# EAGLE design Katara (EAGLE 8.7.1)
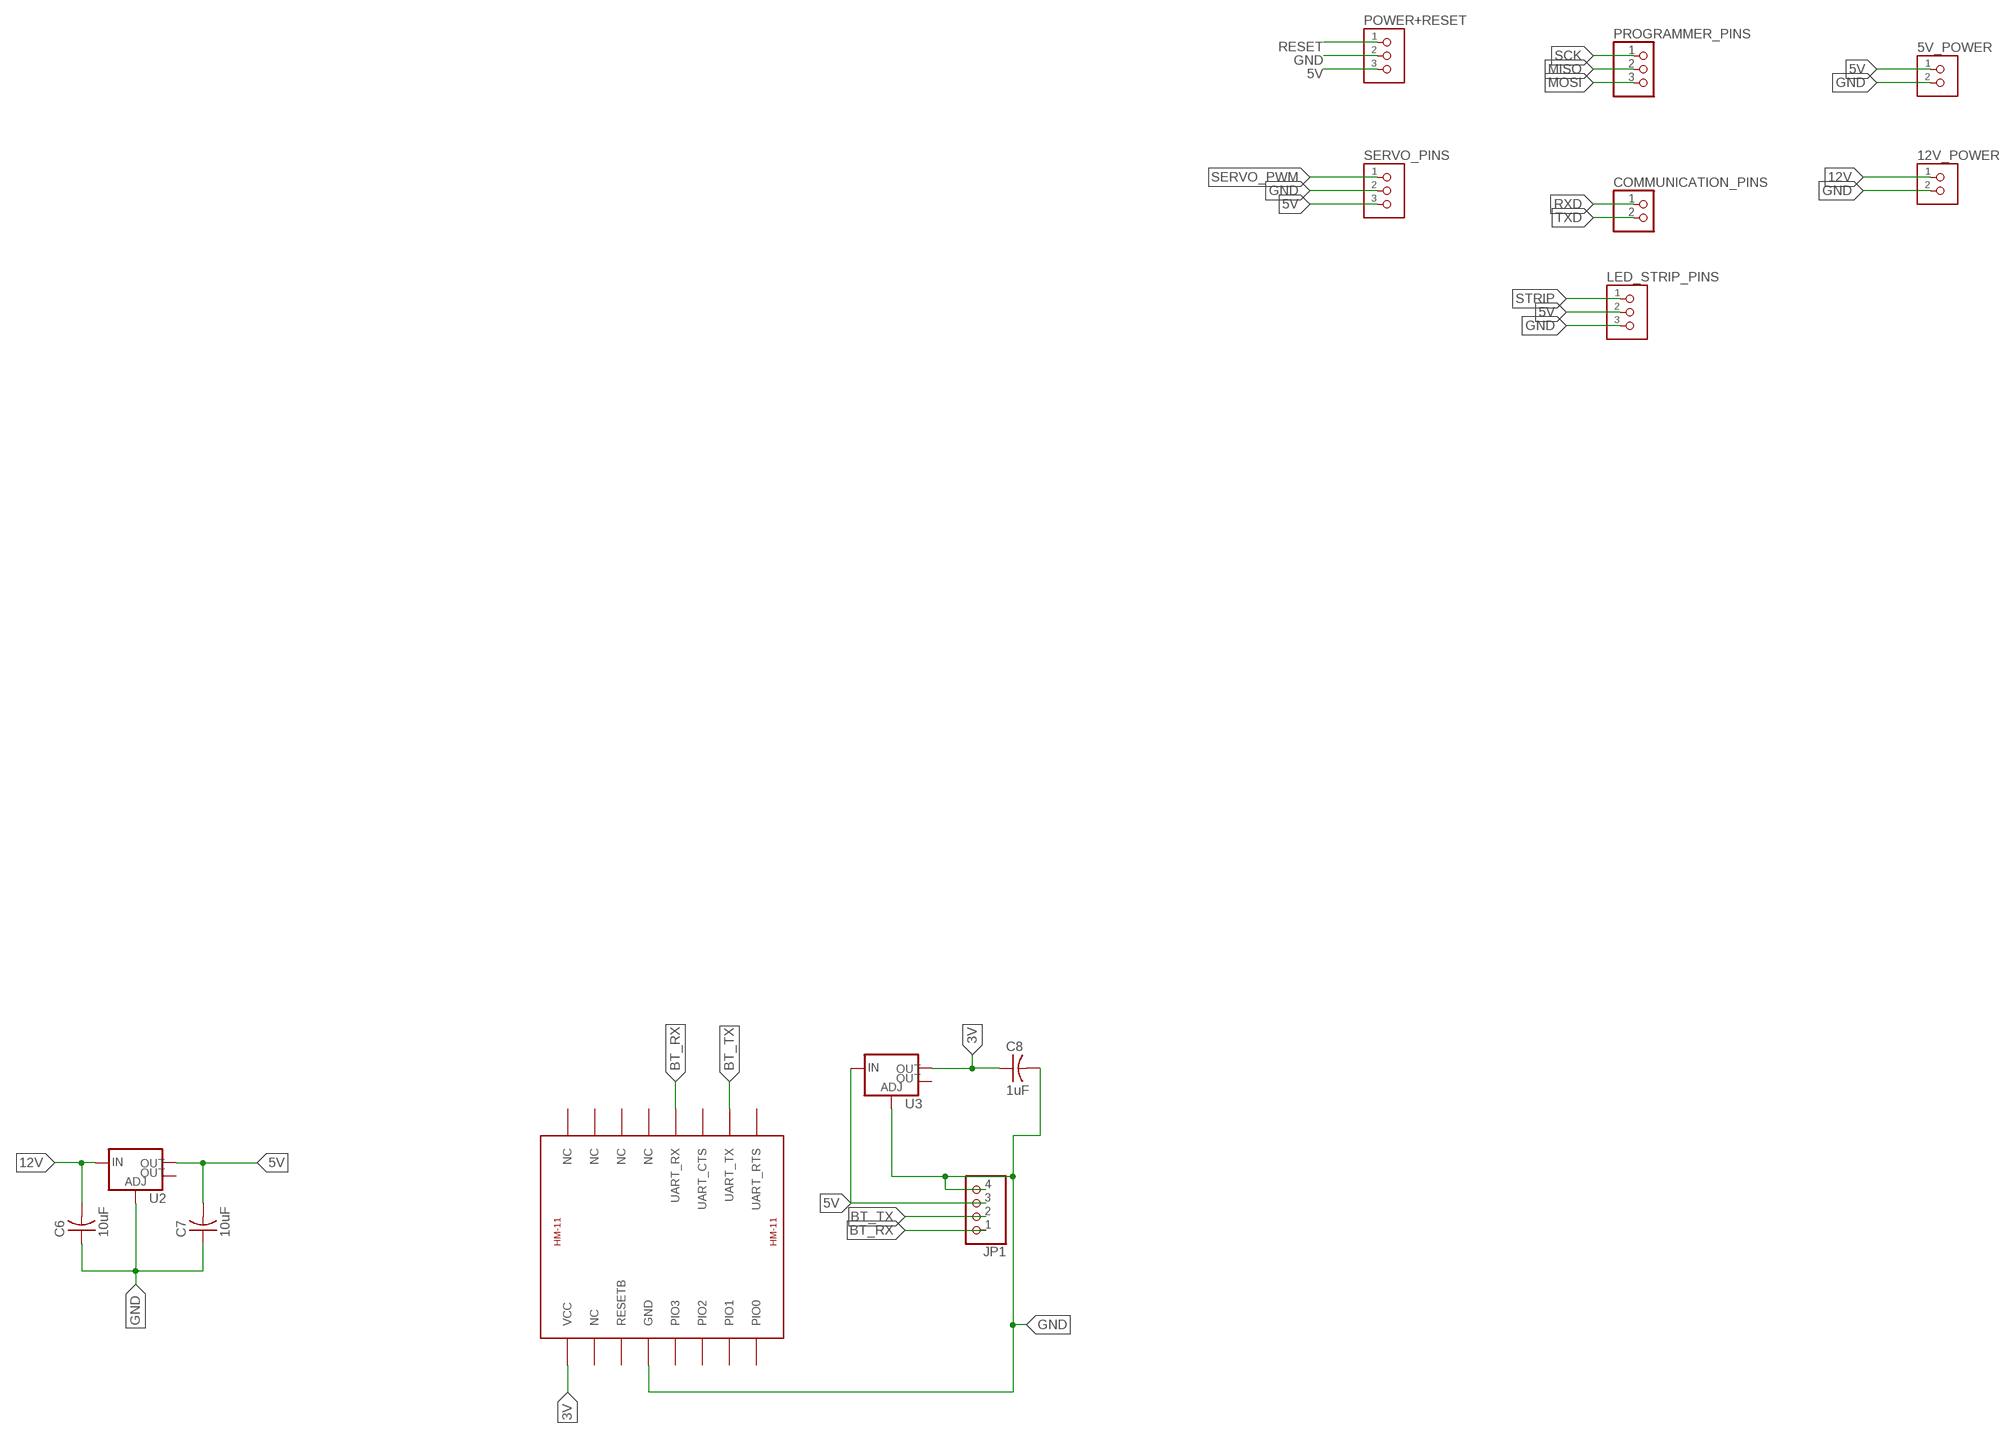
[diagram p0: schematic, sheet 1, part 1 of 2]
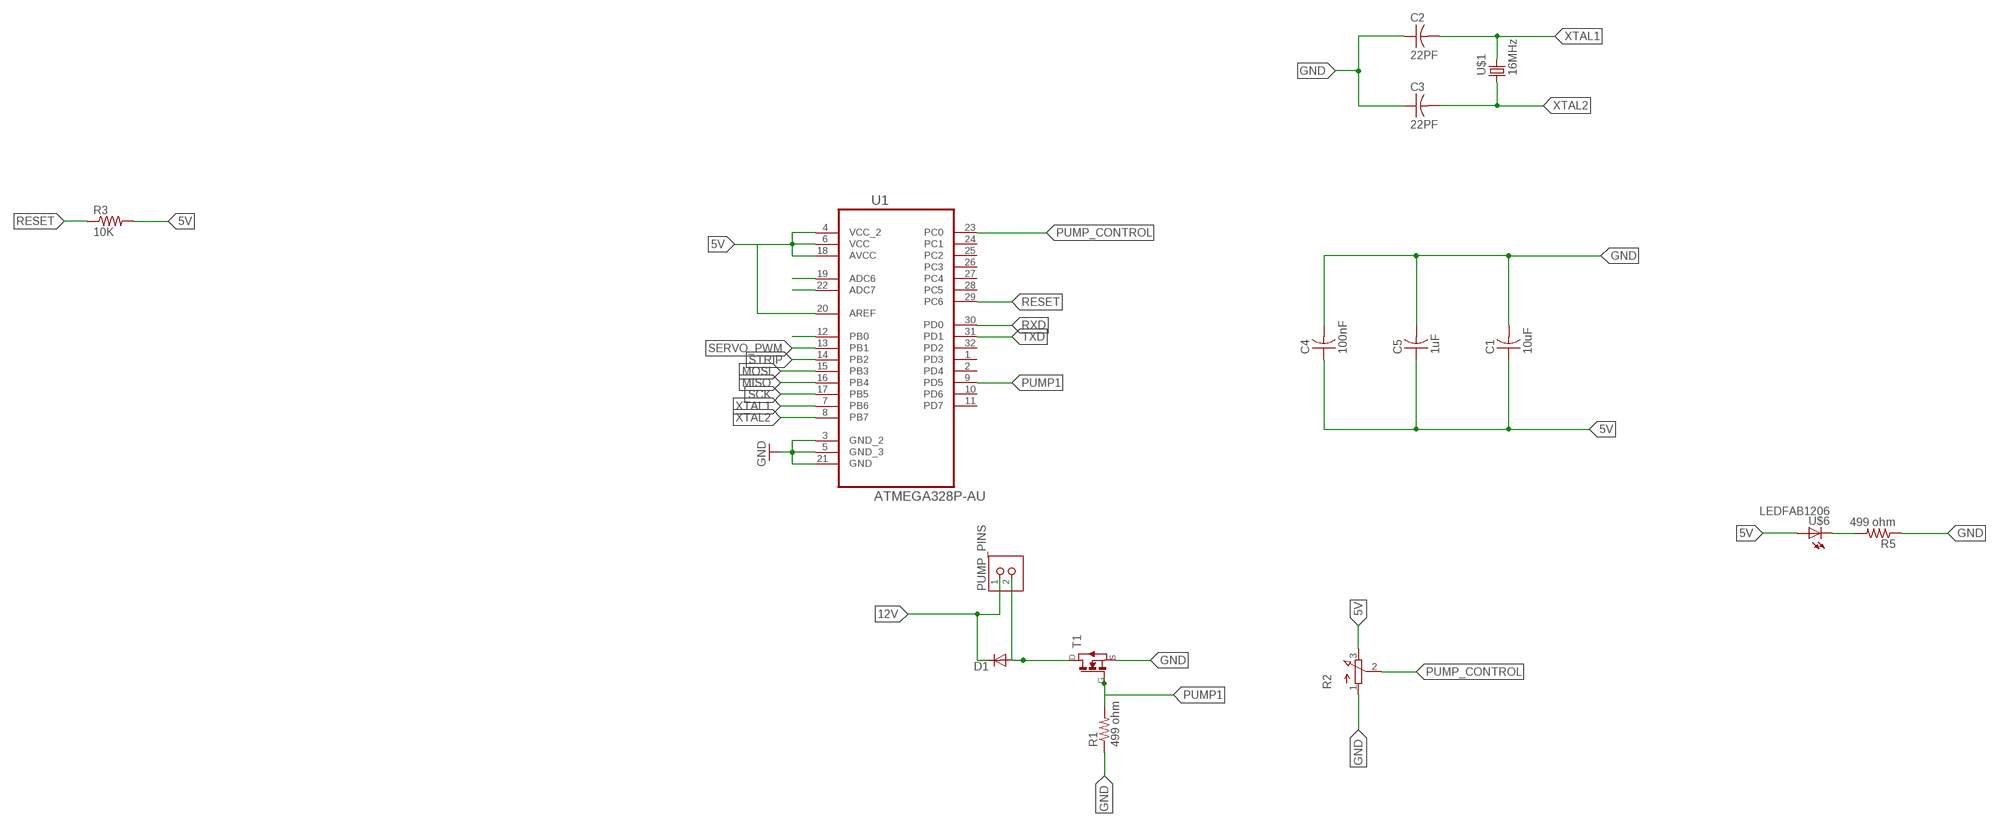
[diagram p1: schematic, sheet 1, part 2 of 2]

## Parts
5V_POWER  TERM-1X02-FABLAB  [ED555DS-2DS]
12V_POWER  TERM-1X02-FABLAB  [ED555DS-2DS]
C1  10uF  CAP-US1206FAB  [C1206FAB]
C2  22PF  CAP-US1206FAB  [C1206FAB]
C3  22PF  CAP-US1206FAB  [C1206FAB]
C4  100nF  CAP-US1206FAB  [C1206FAB]
C5  1uF  CAP-US1206FAB  [C1206FAB]
C6  10uF  CAP-US1206FAB  [C1206FAB]
C7  10uF  CAP-US1206FAB  [C1206FAB]
C8  1uF  CAP-US1206FAB  [C1206FAB]
COMMUNICATION_PINS  PINHD-1X2  [1X02]
D1  DIODE-DO41-10  [DO41-10]
JP1  PINHD-1X4  [1X04]
LED_STRIP_PINS  TERM-1X03'-FABLAB'  [ED555DS-3DS]
POWER+RESET  TERM-1X03'-FABLAB'  [ED555DS-3DS]
PROGRAMMER_PINS  PINHD-1X3  [1X03]
PUMP_PINS  TERM-1X02-FABLAB  [ED555DS-2DS]
R1  499 ohm  RES-US1206FAB  [R1206FAB]
R2  3RP/1610N  [3RP/1610N]
R3  10K  RES-US1206FAB  [R1206FAB]
R5  499 ohm  RES-US1206FAB  [R1206FAB]
SERVO_PINS  TERM-1X03'-FABLAB'  [ED555DS-3DS]
T1  NMOSFETSOT23  [SOT-23]
U1  ATMEGA328P-AU  [QFP80P900X900X120-32N]
U2  V_REG_LM1117SOT223  [SOT223]
U3  V_REG_LM1117SOT223  [SOT223]
U$1  16MHz  CRYSTAL  [2-SMD-5X3MM]
U$2  HM-11  [HM-11]
U$6  LEDFAB1206  [LED1206FAB]

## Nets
3V: C8.1 U3.2(OUT) U$2.VCC
5V: 5V_POWER.1 C1.1 C4.1 C5.1 C7.2 JP1.3 LED_STRIP_PINS.2 POWER+RESET.3 R2.3(E) R3.2 SERVO_PINS.3 U1.4(VCC_2) U1.6(VCC) U1.18(AVCC) U1.20(AREF) U2.2(OUT) U3.3(IN) U$6.1(A)
12V: 12V_POWER.1 C6.2 D1.C PUMP_PINS.1 U2.3(IN)
ADC6: U1.19(ADC6)
ADC7: U1.22(ADC7)
BT_RX: JP1.1 U$2.UART_RX
BT_TX: JP1.2 U$2.UART_TX
D8: U1.12(PB0)
GND: 5V_POWER.2 12V_POWER.2 C1.2 C2.1 C3.1 C4.2 C5.2 C6.1 C7.1 C8.2 JP1.4 LED_STRIP_PINS.3 POWER+RESET.2 R1.1 R2.1(A) R5.1 SERVO_PINS.2 T1.2(S) U1.3(GND_2) U1.5(GND_3) U1.21(GND) U2.1(ADJ) U3.1(ADJ) U$2.GND
MISO: PROGRAMMER_PINS.2 U1.16(PB4)
MOSI: PROGRAMMER_PINS.3 U1.15(PB3)
N$1: D1.A PUMP_PINS.2 T1.1(D)
N$7: R5.2 U$6.2(C)
PUMP1: R1.2 T1.3(G) U1.9(PD5)
PUMP_CONTROL: R2.2(S) U1.23(PC0)
RESET: POWER+RESET.1 R3.1 U1.29(PC6)
RXD: COMMUNICATION_PINS.1 U1.30(PD0)
SCK: PROGRAMMER_PINS.1 U1.17(PB5)
SERVO_PWM: SERVO_PINS.1 U1.13(PB1)
STRIP: LED_STRIP_PINS.1 U1.14(PB2)
TXD: COMMUNICATION_PINS.2 U1.31(PD1)
XTAL1: C2.2 U1.7(PB6) U$1.P$2
XTAL2: C3.2 U1.8(PB7) U$1.P$1
Unconnected: U1.1(PD3) U1.2(PD4) U1.10(PD6) U1.11(PD7) U1.24(PC1) U1.25(PC2) U1.26(PC3) U1.27(PC4) U1.28(PC5) U1.32(PD2) U2.4(OUT) U3.4(OUT) U$2.NC@5(NC) U$2.NC@6(NC) U$2.NC@7(NC) U$2.NC@8(NC) U$2.NC@10(NC) U$2.PIO0 U$2.PIO1 U$2.PIO2 U$2.PIO3 U$2.RESETB U$2.UART_CTS U$2.UART_RTS

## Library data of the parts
5V_POWER 12V_POWER PUMP_PINS = fab:TERM-1X02: 3.5mm terminal block, 2 positions ED555-2DS as found in the fablab inventory.
C1-C8 = fab:CAP-US
COMMUNICATION_PINS = pinhead:PINHD-1X2: PIN HEADER
D1 = diode:DIODE-: DIODE
JP1 = pinhead:PINHD-1X4: PIN HEADER
LED_STRIP_PINS POWER+RESET SERVO_PINS = fab:TERM-1X03: 3.5mm terminal block, 3 positions ED555-3DS as found in the fablab inventory. Made by Zaerc.
PROGRAMMER_PINS = pinhead:PINHD-1X3: PIN HEADER
R1 R3 R5 = fab:RES-US: Resistor (US Symbol)
R2 = pot:3RP/1610N: 16mm Potentiometer one level Source: http://www.alphapotentiometers.net/html/16mm_pot_2.html
T1 = fab:NMOSFET: MOS FET
U1 = ATMEGA328P-AU:ATMEGA328P-AU: 8-bit Microcontroller with In-System Programmable Flash; AVAILABILITY: Good; DESCRIPTION: ATmega Series 20 MHz 32 KB Flash 2 KB SRAM 8-Bit Microcontroller - TQFP-32; MF: Microchip; MP: ATMEGA328P-AU; PACKAGE: TQFP-32 Atmel; PRICE: 2.09 USD
U2 U3 = fab:V_REG_LM1117: Voltage Regulator LM1117 Standard adjustable voltage regulator but in SMD form. Spark Fun Electronics SKU : COM-00595; PROD_ID: VREG-08170
U$1 = fab:CRYSTAL
U$2 = hm-11:HM-11: JNHuaMao HM-11 Bluetooth 4.0 Transceiver based on TI CC2540/CC2541
U$6 = fab:LED: LED

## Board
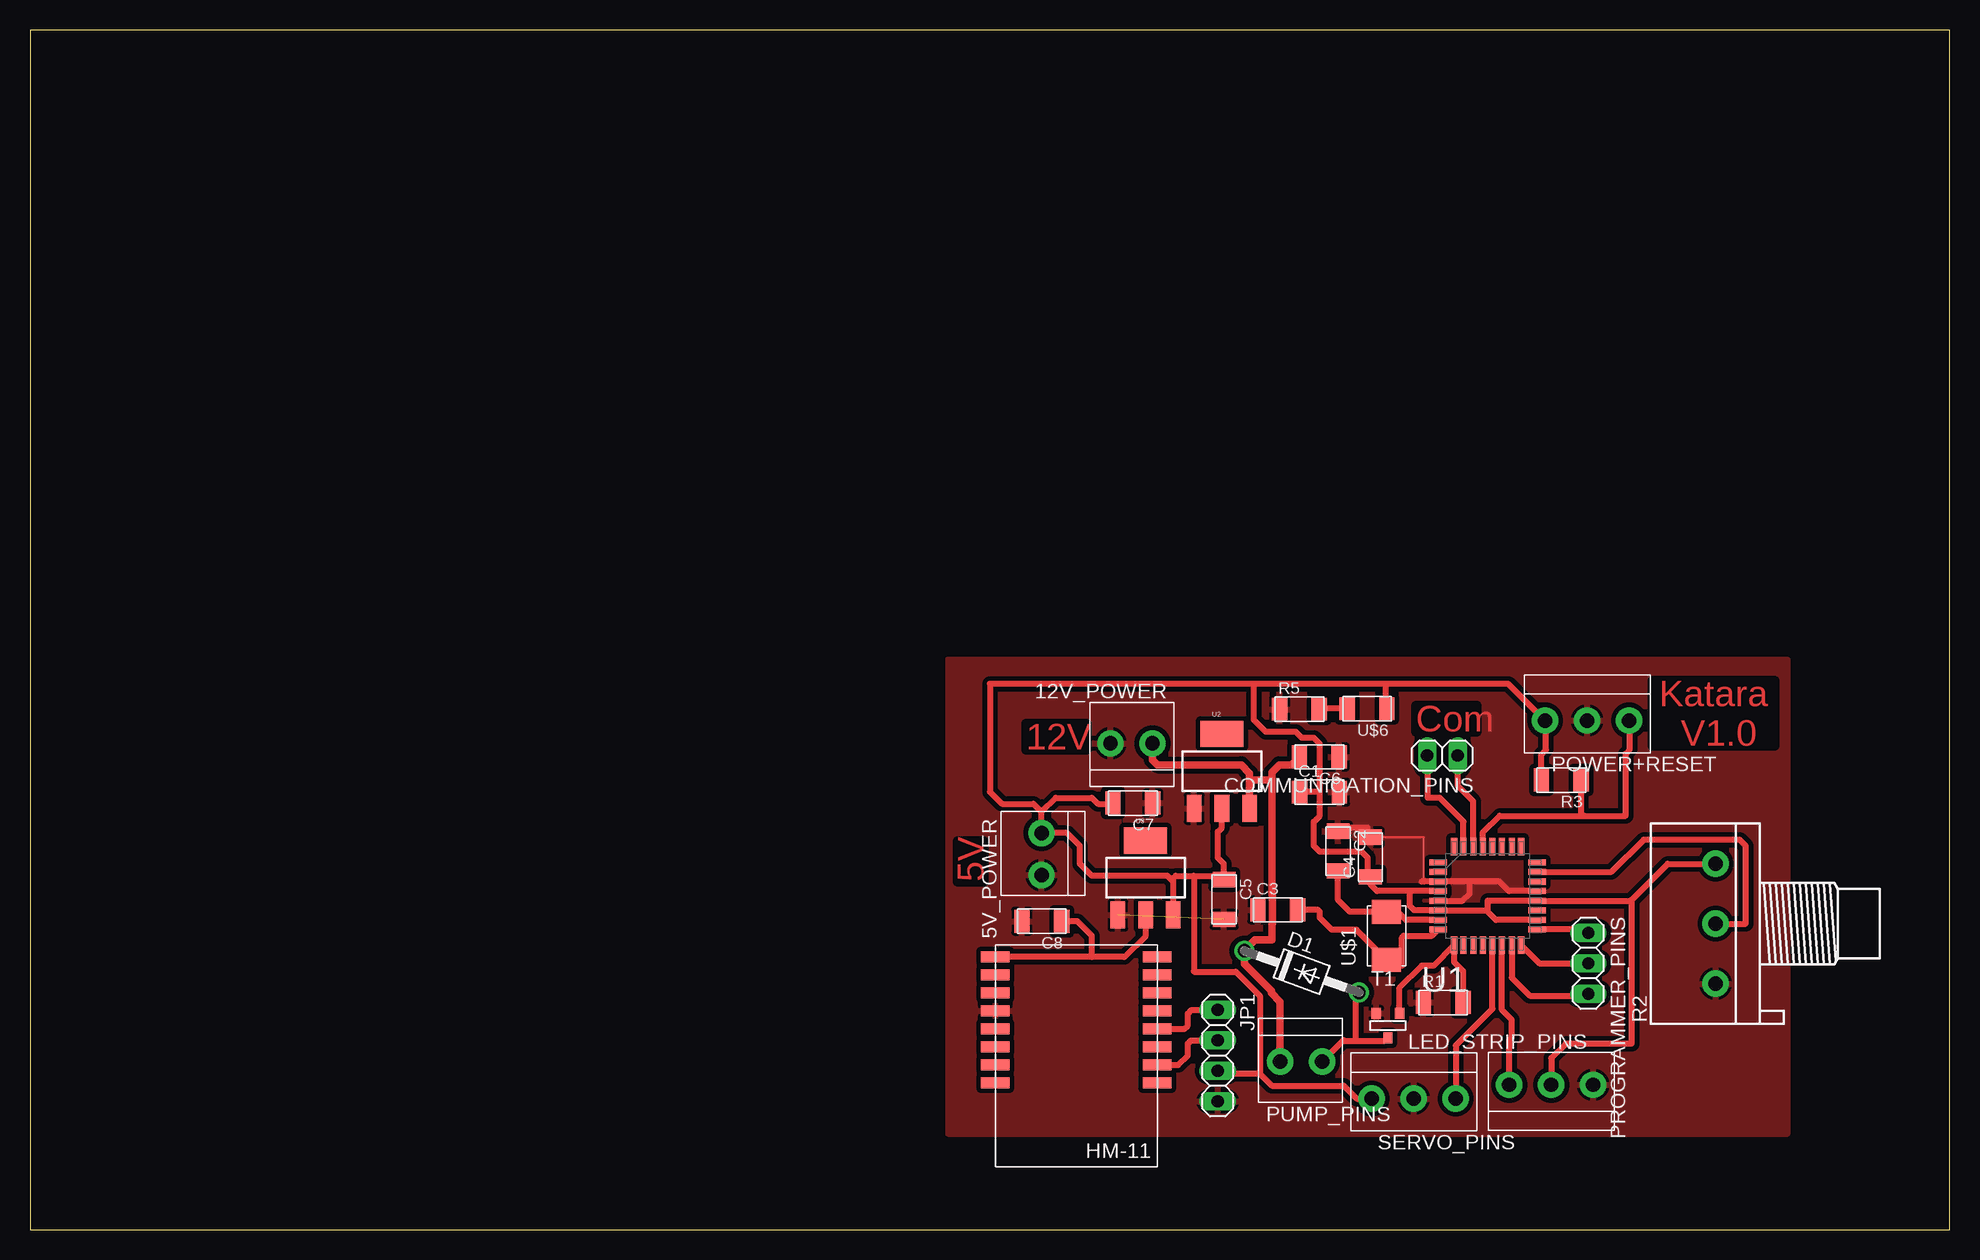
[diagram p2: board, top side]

Size 160 x 100 mm. Coordinates in mm from the lower left corner, seen from the top.
Outline: 0,0 160,0 160,100 0,100 0,0
Copper layers (1*16): Top 0.035mm / dielectric 1.5mm / Bottom 0.035mm
Design rules "default *": minimum track width 6mil, minimum drill 0.35mm, track to track 0.4mm, track to pad 0.25mm, pad to pad 0.1mm, via to via 0.25mm, smd to smd 0.25mm, copper to edge 40mil, drill to drill 6mil, minimum pad ring 10mil, minimum via ring 8mil, stop-mask expansion 4mil, vias tented up to drill 0mil, thermal gap 10mil

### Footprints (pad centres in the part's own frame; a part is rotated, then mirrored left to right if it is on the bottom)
ED555DS-2DS = drill 1.2 pad 2.184: 1 1.8,0; 2 -1.7,0
C1206FAB = smd 1.27 x 1.905: 1 -1.651,0; 2 1.651,0
1X02 = drill 1.016 long: 1 -1.27,0; 2 1.27,0
DO41-10 = drill 1.118: A 5.08,0; C -5.08,0
1X04 = drill 1.016 long: 1 -3.81,0; 2 -1.27,0; 3 1.27,0; 4 3.81,0
ED555DS-3DS = drill 1.2 pad 2.184: 1 -3.5,0; 2 0,0; 3 3.5,0
1X03 = drill 1.016 long: 1 -2.54,0; 2 0,0; 3 2.54,0
R1206FAB = smd 1.27 x 1.905: 1 -1.651,0; 2 1.651,0
3RP/1610N = drill 1.2 pad 2.184: 1 -5,0; 2 0,0; 3 5,0
SOT-23 = smd 0.787 x 0.889: 1 0.025,-1.016; 2 -0.94,1.016; 3 0.991,1.016
QFP80P900X900X120-32N = smd 1.473 x 0.508: 1 -4.115,2.794; 2 -4.115,2.007; 3 -4.115,1.194; 4 -4.115,0.406; 5 -4.115,-0.406; 6 -4.115,-1.194; 7 -4.115,-2.007; 8 -4.115,-2.794; 17 4.115,-2.794; 18 4.115,-2.007; 19 4.115,-1.194; 20 4.115,-0.406; 21 4.115,0.406; 22 4.115,1.194; 23 4.115,2.007; 24 4.115,2.794 | smd 0.508 x 1.473: 9 -2.794,-4.115; 10 -2.007,-4.115; 11 -1.194,-4.115; 12 -0.406,-4.115; 13 0.406,-4.115; 14 1.194,-4.115; 15 2.007,-4.115; 16 2.794,-4.115; 25 2.794,4.115; 26 2.007,4.115; 27 1.194,4.115; 28 0.406,4.115; 29 -0.406,4.115; 30 -1.194,4.115; 31 -2.007,4.115; 32 -2.794,4.115
SOT223 = smd 1.219 x 2.235: 1 -2.311,-3.099; 2 0,-3.099; 3 2.311,-3.099 | smd 3.6 x 2.2: 4 0,3.099
2-SMD-5X3MM = smd 2 x 2.4: P$1 -2,0; P$2 2,0
HM-11 = smd 2.4 x 0.9: GND 6.5,0; NC@5 -7,0; NC@6 -7,-1.5; NC@7 -7,-3; NC@8 -7,-4.5; NC@10 6.5,-3; PIO0 6.5,6; PIO1 6.5,4.5; PIO2 6.5,3; PIO3 6.5,1.5; RESETB 6.5,-1.5; UART_CTS -7,3; UART_RTS -7,6; UART_RX -7,1.5; UART_TX -7,4.5; VCC 6.5,-4.5
LED1206FAB = smd 1.27 x 1.905: 1 -1.651,0; 2 1.651,0

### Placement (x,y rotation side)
5V_POWER  84.32,31.25 90 top
12V_POWER  91.76,40.53 0 top
C1  107.49,36.46 0 top
C2  109.04,31.55 270 top
C3  104.01,26.65 0 top
C4  111.73,31.05 90 top
C5  99.54,27.51 270 top
C6  107.47,39.4 180 top
C7  91.93,35.55 180 top
C8  84.34,25.7 180 top
COMMUNICATION_PINS  117.73,39.51 180 top
D1  106,21.5 340 top
JP1  99,14.5 270 top
LED_STRIP_PINS  126.8,12.06 0 top
POWER+RESET  129.79,42.43 180 top
PROGRAMMER_PINS  129.89,22.19 270 top
PUMP_PINS  106,14 180 top
R1  117.8,18.93 0 top
R2  140.5,25.5 90 top
R3  127.64,37.47 180 top
R5  105.81,43.37 0 top
SERVO_PINS  115.34,10.91 180 top
T1  113.16,17 0 top
U1  121.5,27.81 0 top
U2  99.35,38.21 0 top
U3  92.99,29.32 0 top
U$1  113.07,24.5 90 top
U$2  86.96,18.22 180 top
U$6  111.45,43.42 180 top

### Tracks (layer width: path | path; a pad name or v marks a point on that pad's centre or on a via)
3V
  Top 0.508: U3.2 92.99,24.51 93,24.5 91.22,22.72 88.5,22.72 | 88.5,22.72 U$2.VCC | 88.5,22.72 88.5,24.5 87.3,25.7 C8.1
5V
  Top 0.508: U1.18 122.2,25.8 121.5,26.5 | 121.5,26.5 121.5,27.4 U1.20 133.4,27.4 133.5,27.5 | R2.3 136.5,30.5 133.5,27.5 | 133.5,27.5 133.5,15.5 128,15.5 126.8,14.3 LED_STRIP_PINS.2 | U1.4 115,28.22 | U3.3 95.3,29 | 95.3,29 95.3,29.3 95.5,29.5 97,29.5 | 97,29.5 99.5,29.5 | 95.3,29 94.8,29.5 88.5,29.5 87.5,30.5 87.5,32 86.45,33.05 5V_POWER.1 84.32,34.82 | 102.5,13 103.5,12 109.5,12 110.59,10.91 SERVO_PINS.3 | 97,29.5 97,21.54 97.04,21.5 100.5,21.5 102.5,19.5 102.5,13 | 115,28.22 115,27 115.38,26.62 U1.6 121.38,26.62 121.5,26.5 | 115,28.22 112.28,28.22 111.73,28.77 C4.1 111.5,29.63 111.5,31 111,31.5 107.5,31.5 107,32 107,34 107.5,34.5 107.5,36.5 | 113,45.5 123.22,45.5 126.27,42.45 POWER+RESET.3 126.36,42.36 126.36,40.01 125.98,39.62 R3.2 | 113,45.5 102,45.5 | U$6.1 113,43.52 113,45.5 | C7.2 90.23,35.5 89,35.5 88.5,36 85.5,36 84.32,34.82 | 102.5,13 99.23,13 JP1.3 | 99.5,29.5 99.5,30.5 99,31 99,33.15 99.35,33.5 U2.2 | C5.1 99.54,29.46 99.5,29.5 | 107.5,36.5 107.5,40.5 107,41 106,41 105.5,41.5 103,41.5 102,42.5 102,45.5 | 107.5,36.5 107.46,36.46 C1.1 | 84.32,34.82 83.64,35.5 81,35.5 80,36.5 80,45.5 102,45.5
12V
  Top 0.61: 12V_POWER.1 93.56,39.16 93.98,38.73 100.97,38.73 101.66,38.04 101.66,37.47 | 101.66,37.47 U2.3 | C6.2 105.15,38.73 104.14,38.73 103.5,38.1 103.5,37.47 | 103.5,37.47 103.5,27.88 103.55,27.83 103.55,25.47 103.5,25.42 103.5,24.13 102.12,24.13 D1.C 101.23,22.13 103.46,19.9 103.46,19.73 104.2,18.99 PUMP_PINS.1 | 103.5,37.47 101.66,37.47
BT_RX
  Top 0.508: U$2.UART_RX 96.22,16.72 96.5,17 96.5,18 96.81,18.31 JP1.1
BT_TX
  Top 0.508: U$2.UART_TX 95.72,13.72 96.5,14.5 96.5,15.5 96.77,15.77 JP1.2
GND  (1 unrouted)
  Top 0.152: 116.2,29 116.2,32.7 C4.2
  Top 0.508: U1.21 123.28,28.22 122.5,29 120,29 | 120,29 U1.3 116.2,29 116,29 | U1.5 119.4,27.4 120,28 120,29 | C4.2 111.5,32.93 111.5,33.5 109.34,33.5 C2.1
  pour Top: 76.5,47.5 76.5,8 146.5,8 146.5,47.5 145,47.5
MISO
  Top 0.508: U1.16 125.8,22.19 PROGRAMMER_PINS.2
MOSI
  Top 0.508: U1.15 123.51,20.99 125,19.5 129.74,19.5 PROGRAMMER_PINS.3
N$1
  Top 0.508: PUMP_PINS.2 109.5,15.8 109.5,15.75 110.5,15.75 | 110.5,15.75 112.95,15.75 T1.1 | 110.5,15.75 110.5,18.99 D1.A
N$7
  Top 0.508: U$6.2 107.51,43.42 R5.2
PUMP1
  Top 0.508: R1.2 119.45,21.55 118.71,22.29 U1.9 117.01,22 116,22 114.15,20.15 T1.3
PUMP_CONTROL
  Top 0.508: R2.2 143,25.5 143,32 142.5,32.5 134.5,32.5 131.82,29.82 U1.23
RESET
  Top 0.508: U1.29 121.09,33.09 122.5,34.5 129.29,34.5 | POWER+RESET.1 133.35,42.38 133.35,40.01 133,39.66 133,34.5 129.54,34.5 129.29,34.5 | R3.1 129.29,34.5
RXD
  Top 0.508: U1.30 120.31,35.69 119,37 COMMUNICATION_PINS.1
SCK
  Top 0.508: PROGRAMMER_PINS.1 129.6,25.02 U1.17
SERVO_PWM
  Top 0.508: U1.13 121.91,18.41 118.84,15.34 SERVO_PINS.1
STRIP
  Top 0.508: U1.14 122.69,18.31 123.25,17.75 123.5,17.5 123.5,16 123.3,15.8 LED_STRIP_PINS.1
TXD
  Top 0.508: U1.31 119.49,34.01 117.5,36 116.5,36 116.5,39.47 COMMUNICATION_PINS.2
XTAL1
  Top 0.508: U1.7 114.7,25.8 114,26.5 U$1.P$2 110,26.5 109.04,27.46 C2.2
XTAL2
  Top 0.508: U1.8 116.87,24.5 114.5,24.5 114.37,24.37 114.37,22 U$1.P$1 110.57,25 108.5,25 107.5,26 107.5,26.5 107.35,26.65 C3.2

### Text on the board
Top: Com | 12V | Katara / V1.0 | 5V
